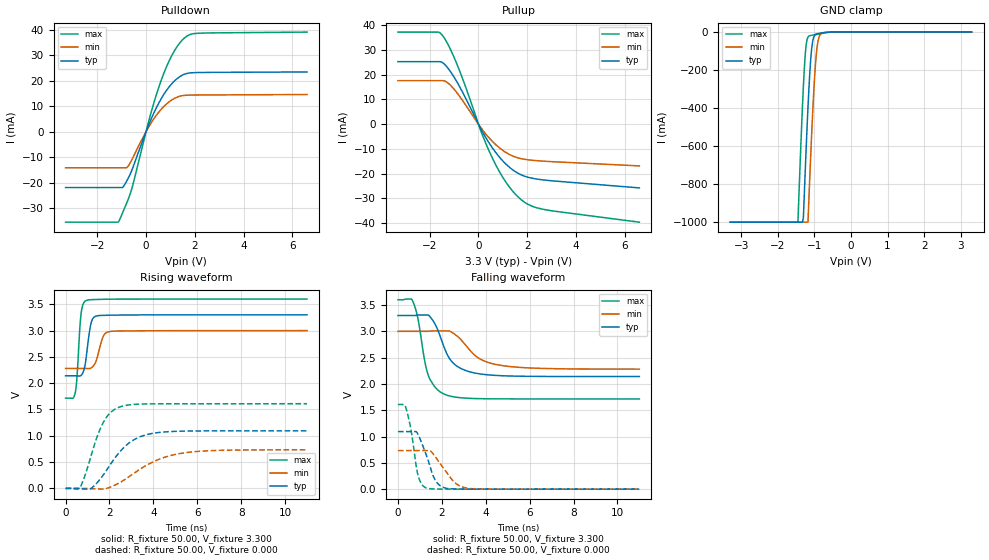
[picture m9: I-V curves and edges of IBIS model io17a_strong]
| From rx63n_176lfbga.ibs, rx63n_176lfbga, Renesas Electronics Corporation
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[Model]   io17a_strong
Model_type   I/O
Polarity   Non-Inverting
Enable   Active-High
Vinl  =   0.660V
Vinh  =   2.640V
Vmeas =   1.650V
Rref  =   882.000
Cref  =   30.00pF
Vref  =   3.300V
| variable   typ   min   max
C_comp   5.360pF   5.360pF   5.360pF
| variable   typ   min   max
[Temperature Range]   45.000   105.000   -40.000
| variable   typ   min   max
[Voltage Range]   3.300V   3.000V   3.600V
| variable   typ   min   max
[Pullup Reference]   3.300V   3.000V   3.600V
| variable   typ   min   max
[Pulldown Reference]   0.000V   0.000V   0.000V
| variable   typ   min   max
[POWER Clamp Reference] 3.300V   3.000V   3.600V
| variable   typ   min   max
[GND Clamp Reference]   0.000V   0.000V   0.000V
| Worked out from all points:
|   slope of the pulldown table from 0 to 0.495 V, typ, clamps not added: 46.2 ohm
|   slope of the pullup table from 0 to 0.495 V, typ, clamps not added: 58.5 ohm
|   GND clamp passes 1 mA (typ) near -0.63 V on its own axis
|   rising waveform, R_fixture 50.00, V_fixture 3.300: 20-80 % time 225ps typ, 291ps min, 167ps max; typ from 2.14 V to 3.3 V
|   rising waveform, R_fixture 50.00, V_fixture 0.000: 20-80 % time 1.28ns typ, 1.87ns min, 821ps max; typ from 0 V to 1.09 V
|   falling waveform, R_fixture 50.00, V_fixture 3.300: 20-80 % time 809ps typ, 1.16ns min, 535ps max; typ from 3.3 V to 2.14 V
|   falling waveform, R_fixture 50.00, V_fixture 0.000: 20-80 % time 557ps typ, 784ps min, 365ps max; typ from 1.09 V to 0 V
[Pulldown]
| io17a_strong Pulldown rx631_rx63n
| Thu Mar 22 17:15:49 2012
| voltage   I(typ)   I(min)   I(max)
-3.3V     -21.93mA   -14.19mA   -35.51mA
-1.125V   -21.93mA   -14.19mA   -35.28mA
-950mV    -21.8mA    -14.19mA   -31.51mA
-725mV    -18.13mA   -13.36mA   -26.35mA
-525mV    -13.67mA   -9.89mA    -20.27mA
200mV     4.744mA    3.297mA    7.31mA
600mV     12.56mA    8.559mA    19.59mA
1.1V      19.27mA    12.7mA     30.64mA
1.375V    21.53mA    13.87mA    34.7mA
1.6V      22.62mA    14.25mA    36.95mA
2.2V      23.2mA     14.39mA    38.62mA
6.6V      23.41mA    14.56mA    39.05mA
[Pullup]
| io17a_strong Pullup rx631_rx63n
| Thu Mar 22 17:15:49 2012
| voltage   I(typ)   I(min)   I(max)
-3.3V     25.27mA    17.59mA    37.22mA
-1.65V    25.27mA    17.59mA    37.22mA
-1.45V    24.69mA    17.59mA    35.55mA
-1.2V     22mA       16.21mA    31.31mA
-900mV    17.41mA    12.94mA    24.72mA
125mV     -2.353mA   -1.734mA   -3.424mA
600mV     -9.977mA   -7.247mA   -14.28mA
1.2V      -16.82mA   -11.88mA   -24.5mA
1.8V      -20.71mA   -14.07mA   -30.92mA
2.2V      -21.87mA   -14.61mA   -33.19mA
2.8V      -22.72mA   -15.06mA   -34.72mA
6.6V      -25.8mA    -16.9mA    -39.66mA
[GND Clamp]
| io17a_strong GNDClamp rx631_rx63n
| Thu Mar 22 17:15:49 2012
| voltage   I(typ)   I(min)   I(max)
-3.3V     -1A        -1A        -1A
-1.45V    -1A        -1A        -998.8mA
-1.325V   -1A        -1A        -385.7mA
-1.3V     -971.8mA   -1A        -281.5mA
-1.25V    -727.5mA   -1A        -116.3mA
-1.175V   -394.3mA   -998.4mA   -26.12mA
-1.15V    -297.8mA   -877.6mA   -21.18mA
-1.075V   -87.77mA   -537.8mA   -16.82mA
-975mV    -12.79mA   -181.3mA   -13.71mA
-900mV    -7.378mA   -46.43mA   -11.41mA
-825mV    -5.325mA   -9.739mA   -8.598mA
3.3V      0A         0A         0A
[POWER Clamp]
| io17a_strong PWRClamp rx631_rx63n
| Thu Mar 22 17:15:49 2012
| voltage   I(typ)   I(min)   I(max)
-3.3V     0A         0A         0A
0V        0A         0A         0A
3.3V      0A         0A         0A
[Ramp]
dV/dt_r   0.657/1.28n   0.440/1.86n   0.966/819.64p
dV/dt_f   0.696/807.69p  0.432/1.17n   1.131/535.34p
R_load = 50.00ohm
[Rising Waveform]
| io17a_strong Rising-High rx631_rx63n
| Thu Mar 22 17:15:49 2012
R_fixture = 50.00
V_fixture = 3.300
V_fixture_min = 3.000
V_fixture_max = 3.600
C_fixture = 0.00pF
| Time   V(typ)   V(min)   V(max)
0s        2.141V     2.28V      1.715V
440ps     2.141V     2.28V      1.819V
515ps     2.141V     2.28V      2.099V
705ps     2.148V     2.28V      3.319V
950ps     2.529V     2.28V      3.575V
1.165ns   3.149V     2.291V     3.588V
1.455ns   3.283V     2.51V      3.593V
1.755ns   3.291V     2.921V     3.596V
2.13ns    3.294V     2.989V     3.598V
11ns      3.3V       3V         3.6V
[Rising Waveform]
| io17a_strong Rising-Low rx631_rx63n
| Thu Mar 22 17:15:49 2012
R_fixture = 50.00
V_fixture = 0.000
C_fixture = 0.00pF
| Time   V(typ)   V(min)   V(max)
0s        0V         0V         0V
665ps     -6mV       0V         22mV
1.16ns    -1mV       -6mV       618mV
1.665ns   226mV      -13mV      1.211V
2.03ns    448mV      23mV       1.435V
2.455ns   688mV      108mV      1.547V
2.965ns   885mV      244mV      1.591V
3.52ns    1V         399mV      1.604V
5.21ns    1.087V     662mV      1.609V
11ns      1.094V     734mV      1.61V
[Falling Waveform]
| io17a_strong Falling-High rx631_rx63n
| Thu Mar 22 17:15:49 2012
R_fixture = 50.00
V_fixture = 3.300
V_fixture_min = 3.000
V_fixture_max = 3.600
C_fixture = 0.00pF
| Time   V(typ)   V(min)   V(max)
0s        3.3V       3V         3.6V
650ps     3.3V       3V         3.595V
900ps     3.309V     3V         3.264V
1.375ns   3.311V     3V         2.173V
1.75ns    3.088V     3.008V     1.912V
2.15ns    2.65V      3.008V     1.799V
2.895ns   2.288V     2.83V      1.736V
3.615ns   2.199V     2.508V     1.721V
4.51ns    2.161V     2.366V     1.716V
11ns      2.141V     2.281V     1.715V
[Falling Waveform]
| io17a_strong Falling-Low rx631_rx63n
| Thu Mar 22 17:15:49 2012
R_fixture = 50.00
V_fixture = 0.000
C_fixture = 0.00pF
| Time   V(typ)   V(min)   V(max)
0s        1.094V     734mV      1.61V
355ps     1.094V     734mV      1.555V
590ps     1.094V     734mV      1.138V
915ps     1.042V     734mV      264mV
1.3ns     639mV      734mV      21mV
1.63ns    229mV      657mV      5mV
1.91ns    70mV       494mV      2mV
2.56ns    5mV        137mV      1mV
3.12ns    2mV        21mV       0V
11ns      0V         0V         0V
